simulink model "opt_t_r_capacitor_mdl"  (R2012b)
settings: Solver=ode45  StartTime=0.0  StopTime=10.0  RelTol=1e-5  AbsTol=1e-5
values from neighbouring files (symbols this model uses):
  MA = a    (= -1)    [opt_t_r_capacitor.m]
  MB = b    (= 1)    [opt_t_r_capacitor.m]
  MC = 1    [opt_t_r_capacitor.m]
  x0 = -3    [opt_t_r_capacitor.m]

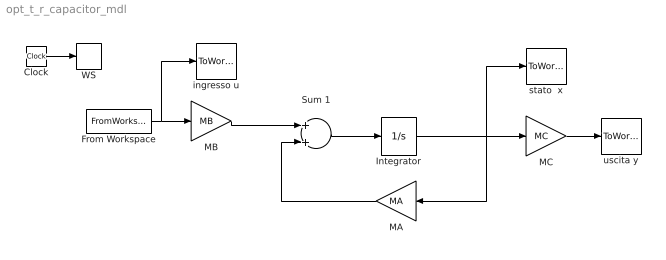
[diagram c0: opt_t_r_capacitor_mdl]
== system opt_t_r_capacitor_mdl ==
  Clock : Clock
  From Workspace : FromWorkspace  VariableName=[T,U]  SampleTime=0
  Integrator : Integrator  InitialCondition=x0
  MA : Gain  Gain=MA  Multiplication=Matrix(K*u)
  MB : Gain  Gain=MB  Multiplication=Matrix(K*u)
  MC : Gain  Gain=MC  Multiplication=Matrix(K*u)
  Sum 1 : Sum
  WS : ToWorkspace  VariableName=t  SampleTime=-1
  ingresso u : ToWorkspace  VariableName=u  SampleTime=-1
  stato  x : ToWorkspace  VariableName=x  SampleTime=-1
  uscita y : ToWorkspace  VariableName=y  SampleTime=-1
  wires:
  MA/1 -> Sum 1/2
  Integrator/1 -> MA/1, MC/1, stato  x/1
  MC/1 -> uscita y/1
  Clock/1 -> WS/1
  Sum 1/1 -> Integrator/1
  MB/1 -> Sum 1/1
  From Workspace/1 -> MB/1, ingresso u/1
